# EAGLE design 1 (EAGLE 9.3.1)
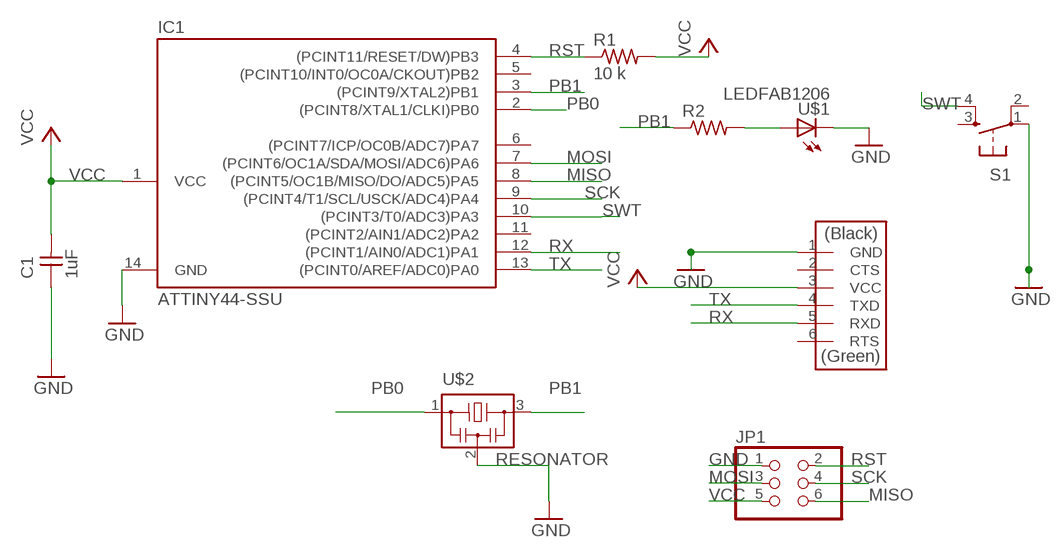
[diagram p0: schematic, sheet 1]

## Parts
C1  1uF  CAP-UNPOLARIZEDFAB  [C1206FAB]
IC1  ATTINY44-SSU  [SOIC14]
JP1  PINHD-2X3-SMD  [2X03SMD]
R1  10 k  RES-US1206FAB  [R1206FAB]
R2  RES-US1206FAB  [R1206FAB]
S1  6MM_SWITCH6MM_SWITCH  [6MM_SWITCH]
U$1  LEDFAB1206  [LED1206FAB]
U$2  RESONATOR  [EFOBM]
U$4  FTDI-SMD-HEADER  [1X06SMD]

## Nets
GND: C1.1 IC1.14(GND) JP1.1 S1.1(P) U$1.2(C) U$2.2 U$4.1(GND)
MISO: IC1.8((PCINT5/OC1B/MISO/DO/ADC5)PA5) JP1.6
MOSI: IC1.7((PCINT6/OC1A/SDA/MOSI/ADC6)PA6) JP1.3
N$2: R2.2 U$1.1(A)
PB0: IC1.2((PCINT8/XTAL1/CLKI)PB0) U$2.1
PB1: IC1.3((PCINT9/XTAL2)PB1) R2.1 U$2.3
RST: IC1.4((PCINT11/RESET/DW)PB3) JP1.2 R1.1
RX: IC1.12((PCINT1/AIN0/ADC1)PA1) U$4.5(RXD)
SCK: IC1.9((PCINT4/T1/SCL/USCK/ADC4)PA4) JP1.4
SWT: IC1.10((PCINT3/T0/ADC3)PA3) S1.4(S1)
TX: IC1.13((PCINT0/AREF/ADC0)PA0) U$4.4(TXD)
VCC: C1.2 IC1.1(VCC) JP1.5 R1.2 U$4.3(VCC)
Unconnected: IC1.5((PCINT10/INT0/OC0A/CKOUT)PB2) IC1.6((PCINT7/ICP/OC0B/ADC7)PA7) IC1.11((PCINT2/AIN1/ADC2)PA2) S1.2(P1) S1.3(S) U$4.2(CTS) U$4.6(RTS)

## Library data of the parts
C1 = fab:CAP-UNPOLARIZED
IC1 = fab:ATTINY44
JP1 = fab:PINHD-2X3-SMD: PIN HEADER
R1 R2 = fab:RES-US: Resistor (US Symbol)
S1 = fab:6MM_SWITCH: OMRON SWITCH
U$1 = fab:LED: LED
U$2 = fab:RESONATOR
U$4 = fab:FTDI-SMD-HEADER

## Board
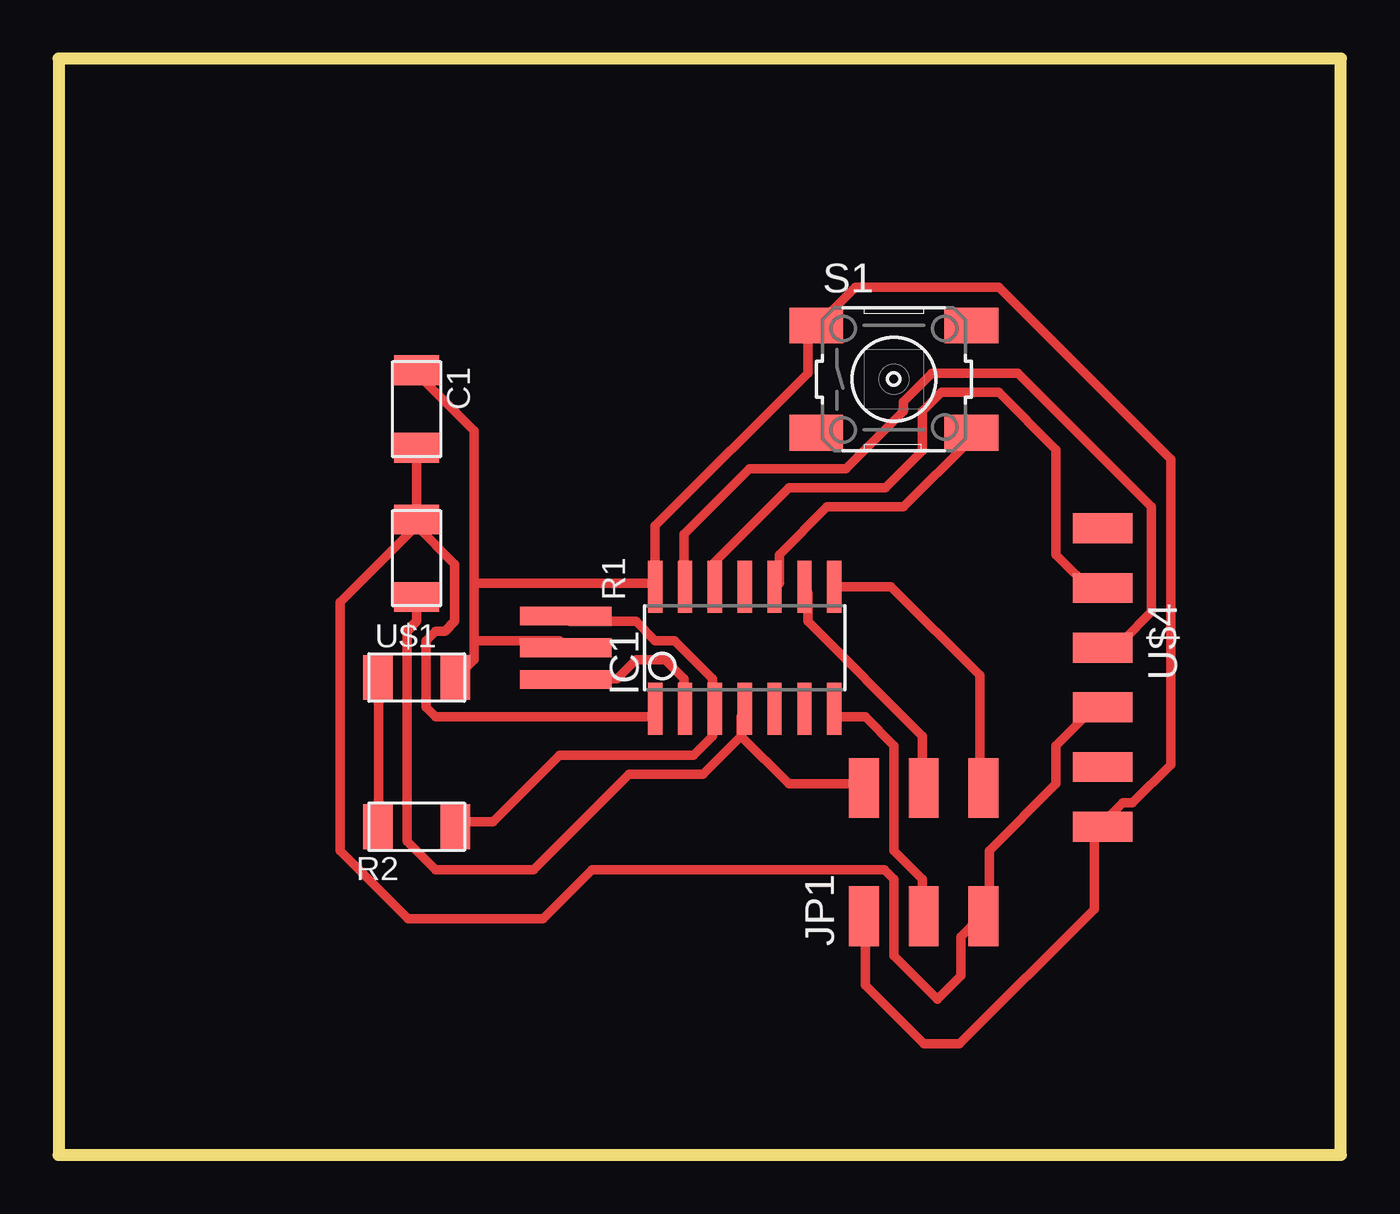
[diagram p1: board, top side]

Size 54.59 x 46.66 mm. Coordinates in mm from the lower left corner, seen from the top.
Outline: 0,0 54.59,0 54.59,46.66 0,46.66 0,0
Copper layers (1*16): Top 0.035mm / dielectric 1.5mm / Bottom 0.035mm
Design rules "default *": minimum track width 16mil, minimum drill 0.35mm, track to track 16mil, track to pad 16mil, pad to pad 16mil, via to via 16mil, smd to smd 16mil, copper to edge 40mil, drill to drill 6mil, minimum pad ring 10mil, minimum via ring 8mil, stop-mask expansion 4mil, vias tented up to drill 0mil, thermal gap 10mil

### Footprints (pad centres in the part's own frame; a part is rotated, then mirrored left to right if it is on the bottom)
C1206FAB = smd 1.27 x 1.905: 1 -1.651,0; 2 1.651,0
SOIC14 = smd 0.61 x 2.21: 1 -3.81,-2.603; 2 -2.54,-2.603; 3 -1.27,-2.603; 4 0,-2.603; 5 1.27,-2.603; 6 2.54,-2.603; 7 3.81,-2.603; 8 3.81,2.603; 9 2.54,2.603; 10 1.27,2.603; 11 0,2.603; 12 -1.27,2.603; 13 -2.54,2.603; 14 -3.81,2.603
2X03SMD = smd 2.54 x 1.27: 1 -2.54,2.54; 2 2.92,2.54; 3 -2.54,0; 4 2.92,0; 5 -2.54,-2.54; 6 2.92,-2.54
R1206FAB = smd 1.27 x 1.905: 1 -1.651,0; 2 1.651,0
6MM_SWITCH = smd 2.286 x 1.524: 1 -3.302,2.286; 2 3.302,2.286; 3 -3.302,-2.286; 4 3.302,-2.286
LED1206FAB = smd 1.27 x 1.905: 1 -1.651,0; 2 1.651,0
EFOBM = smd 0.8 x 3.9: 1 -1.35,0; 2 0,0; 3 1.35,0
1X06SMD = smd 2.54 x 1.27: 1 0,6.35; 2 0,3.81; 3 0,1.27; 4 0,-1.27; 5 0,-3.81; 6 0,-6.35

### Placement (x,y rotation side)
C1  15.24,31.75 270 top
IC1  29.21,21.59 0 top
JP1  36.83,12.7 90 top
R1  15.24,25.4 90 top
R2  15.24,13.97 180 top
S1  35.56,33.02 0 top
U$1  15.24,20.32 0 top
U$2  21.59,21.59 90 top
U$4  44.45,20.32 180 top

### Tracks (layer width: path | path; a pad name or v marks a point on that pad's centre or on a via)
GND
  Top 0.406: JP1.1 34.34,10.11 34.34,7.21 36.83,4.72 38.35,4.72 44.09,10.47 44.09,13.77 U$4.1 44.5,14.17 45.31,14.99 45.72,14.99 47.35,16.61 47.35,29.62 40.03,36.93 33.93,36.93 32.31,35.31 S1.1 31.9,35.31 31.9,33.27 25.4,26.77 25.4,24.33 | 17.68,21.9 17.68,21.08 17.27,20.68 U$1.2 | 17.68,21.9 17.68,24.33 | 17.68,24.33 17.68,30.84 15.24,33.27 C1.1 | 17.68,24.33 25.4,24.33 | 25.4,24.33 IC1.14 | 17.68,21.9 21.34,21.9 U$2.2
MISO
  Top 0.406: IC1.8 35.45,24.19 39.22,20.42 39.22,15.8 JP1.6
MOSI
  Top 0.406: IC1.7 33.12,18.64 34.34,18.64 35.56,17.42 35.56,12.95 36.78,11.73 36.78,10.52 JP1.3
N$2
  Top 0.406: R2.2 13.61,14.17 13.61,20.27 U$1.1
PB0
  Top 0.406: IC1.2 26.62,19.05 26.62,20.27 25.81,21.08 24.59,21.08 23.77,20.27 21.74,20.27 U$2.1
PB1
  Top 0.406: R2.1 17.27,14.17 18.49,14.17 21.34,17.02 27.03,17.02 27.84,17.83 27.84,18.64 IC1.3 27.84,19.05 27.84,20.27 26.21,21.9 25.4,21.9 24.59,22.71 21.74,22.71 U$2.3
RST
  Top 0.406: R1.1 15.24,22.71 14.83,22.3 14.83,13.36 16.05,12.14 20.22,12.14 24.28,16.2 27.43,16.2 29.06,17.83 | 29.06,17.83 29.06,18.64 IC1.4 | 29.06,17.83 31.09,15.8 33.93,15.8 JP1.2
RX
  Top 0.406: IC1.12 27.84,24.33 27.84,25.15 31.09,28.4 35.2,28.4 36.78,29.97 36.78,31.65 37.59,32.46 40.03,32.46 42.47,30.02 42.47,25.55 44.09,23.93 U$4.5
SCK
  Top 0.406: IC1.9 31.9,23.93 31.9,22.71 36.78,17.83 36.78,15.8 JP1.4
SWT
  Top 0.406: IC1.10 30.68,24.33 30.68,25.55 32.71,27.58 35.97,27.58 38.81,30.43 S1.4
TX
  Top 0.406: IC1.13 26.62,24.33 26.62,26.42 29.41,29.21 33.53,29.21 35.97,31.65 35.97,32.05 37.19,33.27 40.84,33.27 46.53,27.58 46.53,23.11 45.31,21.9 44.5,21.9 U$4.4
VCC
  Top 0.406: U$4.3 44.09,19.05 42.47,17.42 42.47,15.8 39.62,12.95 39.62,10.52 JP1.5 39.22,10.11 38.4,9.3 38.4,7.62 37.41,6.63 35.56,8.48 35.56,11.73 35.15,12.14 22.71,12.14 20.62,10.06 14.88,10.06 11.99,12.95 11.99,23.52 15.24,26.77 | C1.2 R1.2 15.24,26.77 | 15.24,26.77 16.87,25.15 16.87,22.71 16.46,22.3 16.05,22.3 15.65,21.9 15.65,19.05 16.05,18.64 25.4,18.64 IC1.1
